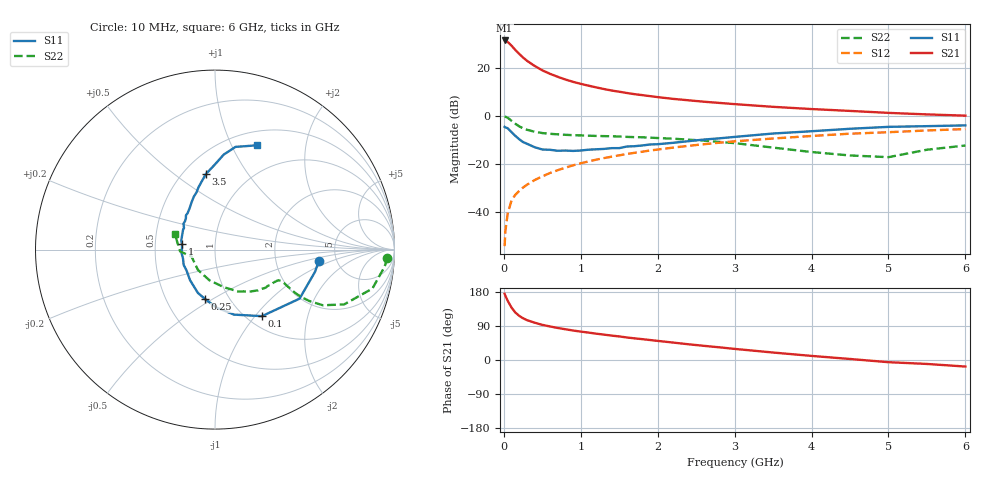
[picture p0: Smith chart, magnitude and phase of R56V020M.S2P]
! SIEMENS Small Signal Semiconductors
! BFR183
! Si NPN RF Bipolar Junction Transistor in SOT23
! VCE = 6 V  IC = 20 mA
! Common Emitter S-Parameters:  May  1996
# GHz  S  MA  R  50
!  f  S11  S21  S12  S22
! GHz  MAG  ANG  MAG  ANG  MAG  ANG  MAG  ANG
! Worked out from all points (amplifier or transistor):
!   36 points, 10 MHz to 6 GHz, reference 50 ohm
!   highest |S21| = 31.3 dB at 10 MHz (marker M1)
!   |S21| within 3 dB of that: start of sweep to 122.7 MHz
!   unconditionally stable (mu >= 1): 605.4 MHz to 2.459 GHz
!   at 250 MHz: K = 0.79, MSG = 27.1 dB, |S12| = -30.0 dB
!   at 1.4 GHz: K = 1.04, MAG = 12.5 dB, |S12| = -17.1 dB
!   at 6 GHz: K = 0.90, MSG = 2.8 dB, |S12| = -5.6 dB
!   S11 on the Smith chart (normalised r, x): 10 MHz: 3.66, -0.67; 100 MHz: 1.16, -1.09; 250 MHz: 0.78, -0.47; 1 GHz: 0.69, +0.05; 3.5 GHz: 0.64, +0.66; 6 GHz: 0.66, +1.26
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0.01  0.5826 -6.0  36.92 174.6  0.0019 90.7  0.9615 -2.7
0.02  0.5711 -12.4  36.25 169.6  0.0039 84.1  0.9496 -5.8
0.05  0.5448 -30.1  34.38 156.3  0.0091 77.5  0.9035 -13.9
0.1  0.4538 -54.8  28.72 138.3  0.0171 71.8  0.7816 -23.0
0.15  0.3774 -73.7  23.34 125.2  0.0225 68.4  0.6761 -27.3
0.2  0.322 -88.8  19.35 116.5  0.027 68.5  0.5981 -28.6
0.25  0.2815 -101.1  16.25 110.1  0.0317 68.4  0.5436 -28.8
0.3  0.2596 -111.5  13.95 105.3  0.0362 69.0  0.508 -28.4
0.4  0.2199 -129.2  10.87 98.5  0.0454 69.9  0.4616 -27.1
0.5  0.1968 -143.6  8.808 92.7  0.0541 71.0  0.4332 -26.1
0.6  0.1942 -154.0  7.441 88.5  0.0637 71.1  0.4179 -25.6
0.7  0.1851 -164.4  6.451 84.5  0.0729 71.3  0.4077 -25.5
0.8  0.1873 -173.9  5.666 81.1  0.0822 70.5  0.3984 -25.6
1  0.1875 170.1  4.597 74.9  0.1015 69.9  0.3871 -26.6
1.1  0.195 164.3  4.216 72.3  0.111 69.3  0.3822 -27.7
1.3  0.2023 153.7  3.588 67.0  0.1301 67.4  0.3741 -29.6
1.6  0.2272 140.6  2.962 59.4  0.1584 64.9  0.3606 -33.6
2.2  0.2712 121.3  2.237 46.0  0.2156 58.6  0.331 -43.3
3.5  0.4239 96.9  1.526 19.7  0.3337 42.5  0.2156 -76.5
4.5  0.5321 84.7  1.254 2.7  0.4203 30.1  0.1478 -130.1
5.5  0.6035 72.9  1.061 -10.4  0.491 18.6  0.1947 -177.0
6  0.6265 68.1  0.999 -17.3  0.5249 11.1  0.2383 159.3
